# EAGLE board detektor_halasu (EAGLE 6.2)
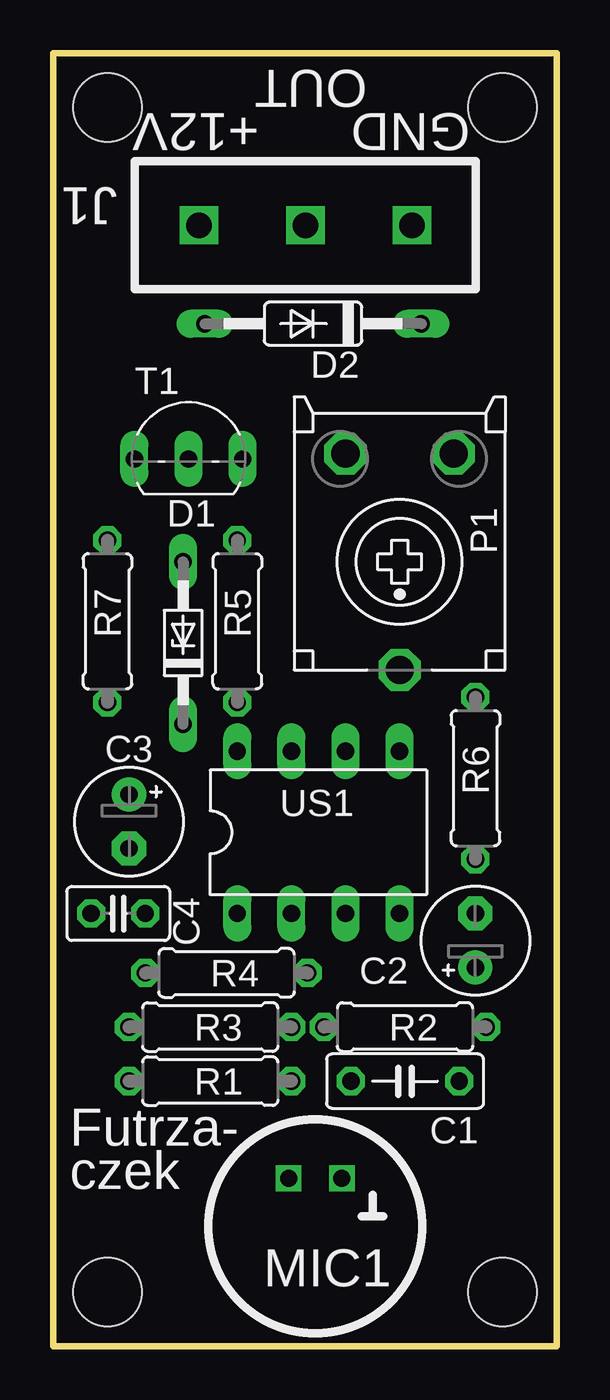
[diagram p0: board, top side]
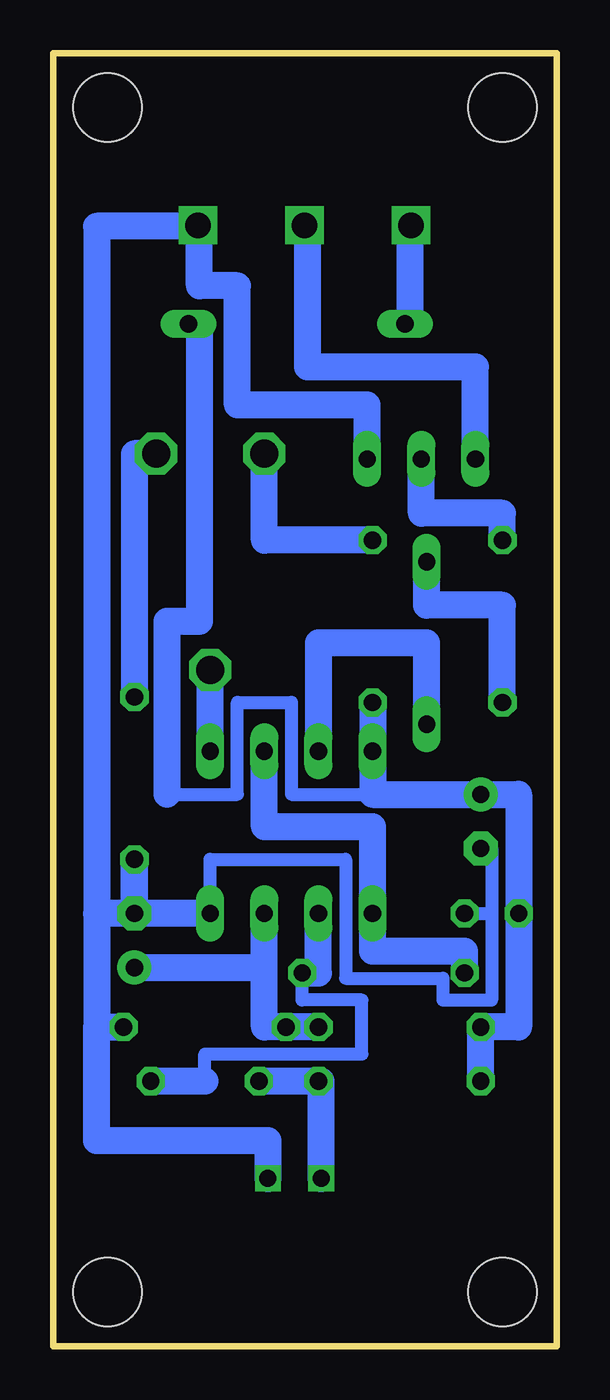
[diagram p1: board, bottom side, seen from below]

Size 23.62 x 60.71 mm. Coordinates in mm from the lower left corner, seen from the top.
Outline: 23.62,60.71 23.62,0 0,0 0,60.71 23.62,60.71
Copper layers (1*16): Top 0.035mm / dielectric 1.5mm / Bottom 0.035mm
Design rules: minimum track width 10mil, minimum drill 24mil, track to track 8mil, track to pad 8mil, pad to pad 8mil, via to via 8mil, smd to smd 8mil, copper to edge 40mil, drill to drill 8mil, minimum pad ring 10mil, minimum via ring 8mil, stop-mask expansion 4mil, vias tented up to drill 0mil, thermal gap 10mil
Holes 3.2 mm at 2.54,58.17 21.08,58.17 2.54,2.54 21.08,2.54

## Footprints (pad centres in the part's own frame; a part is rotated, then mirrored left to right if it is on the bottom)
C050-025X075 = drill 0.813 octagon: 1 -2.54,0; 2 2.54,0
E2,5-5 = drill 0.813 pad 1.6: + -1.27,0 | drill 0.813 pad 1.6 octagon: - 1.27,0
C025-025X050 = drill 0.813 octagon: 1 -1.27,0; 2 1.27,0
DO34Z7 = drill 0.813 long: A 3.81,0; C -3.81,0
DO35-10 = drill 0.813 long: A 5.08,0; C -5.08,0
ECP10S = drill 1.321 octagon: A -2.54,-5.08; E 2.54,-5.08; S 0,5.08
0207/7 = drill 0.813 octagon: 1 -3.81,0; 2 3.81,0
TO92- = drill 0.813 long: 1 2.54,0; 2 0,0; 3 -2.54,0
DIL08 = drill 0.813 long: 1 -3.81,-3.81; 2 -1.27,-3.81; 3 1.27,-3.81; 4 3.81,-3.81; 5 3.81,3.81; 6 1.27,3.81; 7 -1.27,3.81; 8 -3.81,3.81

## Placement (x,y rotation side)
C1  [C050-025X075]  16.51,12.45 180 top
C2  [E2,5-5]  19.81,19.05 90 top
C3  [E2,5-5]  3.56,24.64 270 top
C4  [C025-025X050]  3.05,20.32 0 top
D1  [DO34Z7]  6.1,33.02 90 top
D2  [DO35-10]  12.19,48.01 180 top
P1  [ECP10S]  16.26,36.83 180 top
R1  [0207/7]  7.37,12.45 180 top
R2  [0207/7]  16.51,14.99 180 top
R3  [0207/7]  7.37,14.99 180 top
R4  [0207/7]  8.13,17.53 180 top
R5  [0207/7]  8.64,34.04 270 top
R6  [0207/7]  19.81,26.67 270 top
R7  [0207/7]  2.54,34.04 270 top
T1  [TO92-]  6.35,41.66 0 top
US1  [DIL08]  12.45,24.13 0 top

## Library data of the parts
C1-C4 R1-R7 = rcl
D1 D2 = diode
P1 = pot
T1 = transistor-npn
US1 = 40xx

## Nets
S$3: R4.2 US1.1 US1.6
S$4: C4.2
S$6: R7.2
S$7: R3.1
S$9: C2.+
S$10: R1.1
S$11: R4.1 US1.2
S$13: P1.A R6.1
S$15: R2.1 R6.2 US1.4
S$16: P1.S US1.5
S$17: P1.E R5.1
S$21: D2.A
S$22: D2.C R1.2 R3.2
S$23: R7.1 T1.2

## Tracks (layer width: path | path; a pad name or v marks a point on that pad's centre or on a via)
S$1  (via drill 0.8)
  other vias: 11.05,7.88
S$2  (via drill 0.8)
  other vias: 13.55,7.88
S$3
  Bottom 1.27: R4.2 4.32,18.54 8.64,18.54 US1.1 8.64,24.38 13.72,24.38 US1.6
S$4
  Bottom 0.61: C4.2 3.05,20.32
S$5
  Bottom 1.27: 6.1,28.7 6.1,33.02 11.18,33.02 11.18,27.69
S$6
  Bottom 1.27: R7.2 2.54,34.8 6.1,34.8 6.1,37.08
S$7
  Bottom 1.27: R3.1 13.72,14.99 13.72,20.57
S$9
  Bottom 1.27: C2.+ 13.97,17.78
S$10
  Bottom 1.27: R1.1 13.97,12.45
S$11
  Bottom 0.61: 16.51,12.45 16.51,13.72 9.14,13.72 9.14,16.26 11.94,16.26 R4.1
  Bottom 1.27: 16.51,12.45 19.05,12.45 | R4.1 11.18,17.53 US1.2
S$12
  Bottom 1.27: 11.05,7.87 11.05,12.45
S$13
  Bottom 1.27: P1.A 19.81,41.91 R6.1
S$14
  Bottom 1.27: 19.81,20.57 19.81,22.61
S$15
  Bottom 0.61: US1.4 16.26,22.86 9.91,22.86 9.91,17.27 5.33,17.27 5.33,16.26 3.05,16.26 3.05,23.37 3.56,23.37
  Bottom 1.27: 13.54,7.87 13.54,9.65 21.59,9.65 21.59,14.99 | US1.4 19.81,20.32 | 19.81,20.32 21.59,20.32 | 21.59,20.32 21.59,14.99 | 21.59,14.99 R2.1 | R6.2 19.81,20.32 | 17.02,52.58 21.59,52.58 21.59,20.32
S$16
  Bottom 1.27: US1.5 P1.S
S$17
  Bottom 1.27: R5.1 13.72,37.85 P1.E
S$18  (via drill 1.2)
  other vias: 6.83,52.63
S$19  (via drill 1.2)
  other vias: 11.83,52.63
S$20  (via drill 1.2)
  other vias: 16.83,52.63
S$21
  Bottom 1.27: D2.A 6.86,48.01 6.86,52.58
S$22
  Bottom 0.61: 18.29,25.91 14.99,25.91 14.99,30.23 12.45,30.23 12.45,25.91 8.64,25.91
  Bottom 1.27: D2.C 16.76,48.01 16.76,34.04 18.29,34.04 18.29,25.91 | R1.2 R3.2 1.78,14.99 1.78,25.91 8.64,25.91 8.64,30.23
S$23
  Bottom 1.27: R7.1 2.54,39.12 6.35,39.12 T1.2
S$24
  Bottom 1.27: 8.89,41.15 8.89,44.2 14.99,44.2 14.99,49.78 16.76,49.78 16.76,52.58
S$25
  Bottom 1.27: 3.81,41.91 3.81,45.97 11.68,45.97 11.68,52.58

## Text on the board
tNames: OUT | +12V | GND | J1 | Futrza- | czek | MIC1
